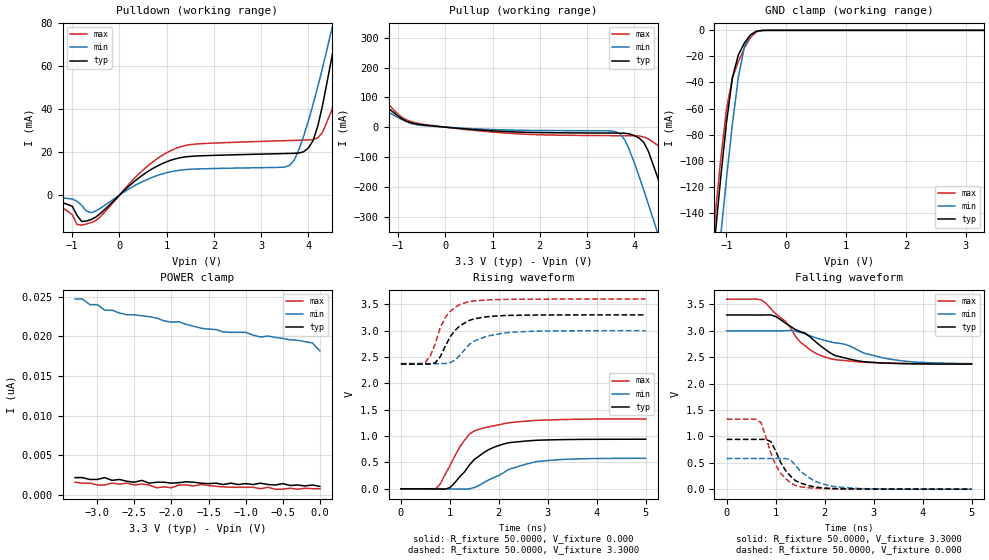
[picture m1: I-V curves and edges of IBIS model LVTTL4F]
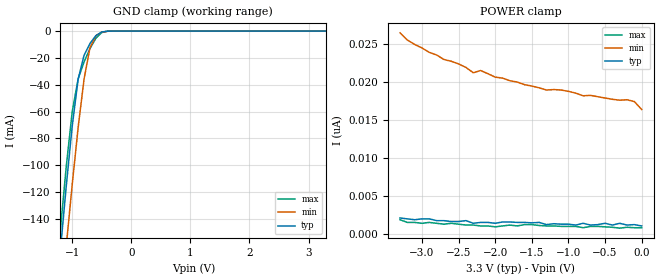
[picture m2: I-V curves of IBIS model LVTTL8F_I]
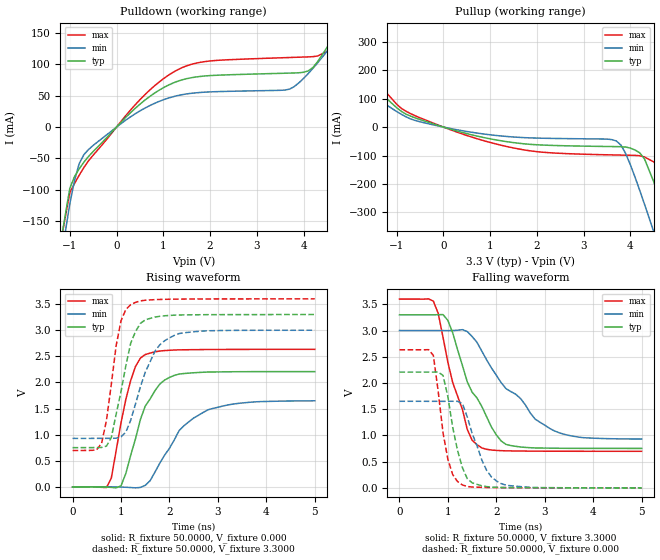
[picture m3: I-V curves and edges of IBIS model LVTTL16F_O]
| Xilinx Virtex IBIS File
[IBIS ver]   2.1
[File name]   virtex.ibs
[File Rev]   1.1
[Date]   Mar. 16, 2001
[Source]   Hspice simulations (23e: TT, SS, FF)
[Notes]   Xilinx IBIS model for Virtex I/O
   The package models are provided for BG432, BG352, BG256,
   BG560, HQ240, PQ240, CS144, TQ144, FG256, FG456, FG676
   and FG680 package types, with BG432 being selected as
   a default. Please make your own selection of the packages
   by commenting out the unused ones.
   COMMENTS: Models include process corners for MIN and MAX.
[Disclaimer] The data in this model is derived from SPICE simulations using
   modeling information extracted from the target process. While
   a great deal of care has been taken to provide information
   that is accurate, this model is considered preliminary as it
   has not been verified by actual silicon measurement. Treat the
   data in this model as preliminary until actual silicon
   verification is performed.
[Copyright]   Copyright 1998, Xilinx Inc., All rights reserved
|   Component Virtex
|   >>> Make Your Selection of the Package type Below <<<
[Component]   VIRTEX
[Manufacturer]   Xilinx Inc.
[Package]
| For Package type BG432:
| variable   typ   min   max
R_pkg   0.2500   0.1600   0.3500
L_pkg   4.9000nH   2.4000nH   7.4000nH
C_pkg   1.0500pF   0.8000pF   1.3000pF
| For Package type BG352:
| variable   typ   min   max
|R_pkg   0.2340   0.1640   0.3040
|L_pkg   6.5500nH   3.8000nH   9.3000nH
|C_pkg   1.0200pF   0.7300pF   1.3100pF
| For Package type BG256:
| variable   typ   min   max
|R_pkg   0.1780   0.1700   0.1850
|L_pkg   4.5000nH   2.3000nH   6.7000nH
|C_pkg   1.4500pF   1.2000pF   1.7000pF
| For Package type BG560:
| variable   typ   min   max
|R_pkg   0.2240   0.1480   0.3000
|L_pkg   5.4500nH   2.0000nH   8.9000nH
|C_pkg   1.0500pF   0.5000pF   1.6000pF
| For Package type HQ240:
| variable   typ   min   max
|R_pkg   0.208   0.202   0.215
|L_pkg   13.2nH   9.00nH   17.3nH
|C_pkg   2.25pF   2.00pF   2.50pF
| For Package type PQ240:
| variable   typ   min   max
|R_pkg   0.208   0.205   0.218
|L_pkg   18.9nH   11.9nH   25.8nH
|C_pkg   1.60pF   1.30pF   1.90pF
| For Package type CS144:
| variable   typ   min   max
|R_pkg   0.116   0.078   0.153
|L_pkg   3.55nH   1.5nH   5.60nH
|C_pkg   0.60pF   0.5pF   0.7pF
| For Package type TQ144:
| variable   typ   min   max
|R_pkg   0.118   0.112   0.124
|L_pkg   9.50nH   5.7nH   13.3nH
|C_pkg   0.95pF   0.8pF   1.1pF
| For Package type FG256:
| variable   typ   min   max
|R_pkg   0.141   0.095   0.187
|L_pkg   4.25nH   1.7nH   6.80nH
|C_pkg   0.75pF   0.60pF   0.90pF
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[Pin]  signal_name   model_name   R_pin   L_pin   C_pin
1   LVCMOS2   LVCMOS2
1I   LVCMOS2_I   LVCMOS2_I
1O   LVCMOS2_O   LVCMOS2_O
2   LVTTL2F   LVTTL2F
2I   LVTTL2F_I   LVTTL2F_I
2O   LVTTL2F_O   LVTTL2F_O
3   LVTTL4F   LVTTL4F
3I   LVTTL4F_I   LVTTL4F_I
3O   LVTTL4F_O   LVTTL4F_O
4   LVTTL6F   LVTTL6F
4I   LVTTL6F_I   LVTTL6F_I
4O   LVTTL6F_O   LVTTL6F_O
5   LVTTL8F   LVTTL8F
5I   LVTTL8F_I   LVTTL8F_I
5O   LVTTL8F_O   LVTTL8F_O
6   LVTTL12F   LVTTL12F
6I   LVTTL12F_I   LVTTL12F_I
6O   LVTTL12F_O   LVTTL12F_O
7   LVTTL16F   LVTTL16F
7I   LVTTL16F_I   LVTTL16F_I
7O   LVTTL16F_O   LVTTL16F_O
8   LVTTL24F   LVTTL24F
8I   LVTTL24F_I   LVTTL24F_I
8O   LVTTL24F_O   LVTTL24F_O
9   LVTTL2S   LVTTL2S
9I   LVTTL2S_I   LVTTL2S_I
9O   LVTTL2S_O   LVTTL2S_O
10   LVTTL4S   LVTTL4S
10I   LVTTL4S_I   LVTTL4S_I
10O   LVTTL4S_O   LVTTL4S_O
11   LVTTL6S   LVTTL6S
11I   LVTTL6S_I   LVTTL6S_I
11O   LVTTL6S_O   LVTTL6S_O
12   LVTTL8S   LVTTL8S
12I   LVTTL8S_I   LVTTL8S_I
12O   LVTTL8S_O   LVTTL8S_O
13   LVTTL12S   LVTTL12S
13I   LVTTL12S_I   LVTTL12S_I
13O   LVTTL12S_O   LVTTL12S_O
14   LVTTL16S   LVTTL16S
14I   LVTTL16S_I   LVTTL16S_I
14O   LVTTL16S_O   LVTTL16S_O
15   LVTTL24S   LVTTL24S
15I   LVTTL24S_I   LVTTL24S_I
15O   LVTTL24S_O   LVTTL24S_O
16   HSTL1   HSTL1
16I   HSTL1_I   HSTL1_I
16O   HSTL1_O   HSTL1_O
17   HSTL3   HSTL3
17I   HSTL3_I   HSTL3_I
17O   HSTL3_O   HSTL3_O
18   HSTL4   HSTL4
18I   HSTL4_I   HSTL4_I
18O   HSTL4_O   HSTL4_O
19   SSTL2C1   SSTL2C1
19I   SSTL2C1_I   SSTL2C1_I
19O   SSTL2C1_O   SSTL2C1_O
20   SSTL2C2   SSTL2C2
20I   SSTL2C2_I   SSTL2C2_I
20O   SSTL2C2_O   SSTL2C2_O
21   SSTL3C1   SSTL3C1
21I   SSTL3C1_I   SSTL3C1_I
21O   SSTL3C1_O   SSTL3C1_O
22   SSTL3C2   SSTL3C2
22I   SSTL3C2_I   SSTL3C2_I
22O   SSTL3C2_O   SSTL3C2_O
23   CTT   CTT
23I   CTT_I   CTT_I
23O   CTT_O   CTT_O
24   AGP   AGP
24I   AGP_I   AGP_I
24O   AGP_O   AGP_O
25   GTL   GTL
25I   GTL_I   GTL_I
25O   GTL_O   GTL_O
26   GTL-PLUS   GTL-PLUS
26I   GTL-PLUS_I   GTL-PLUS_I
26O   GTL-PLUS_O   GTL-PLUS_O
27   PCI33M5V   PCI33M5V
27I   PCI33M5V_I   PCI33M5V_I
27O   PCI33M5V_O   PCI33M5V_O
28   PCI33M3V   PCI33M3V
28I   PCI33M3V_I   PCI33M3V_I
28O   PCI33M3V_O   PCI33M3V_O
29   PCI66M3V   PCI66M3V
29I   PCI66M3V_I   PCI66M3V_I
29O   PCI66M3V_O   PCI66M3V_O
PGND   GND   GND
VCCO   VCCO   POWER
| Models and submodels in the file (87): LVCMOS2 (I/O), LVCMOS2_I (Input), LVCMOS2_O (Output), LVTTL2F (I/O), LVTTL2F_I (Input), LVTTL2F_O (Output), LVTTL4F (I/O), LVTTL4F_I (Input), LVTTL4F_O (Output), LVTTL6F (I/O), LVTTL6F_I (Input), LVTTL6F_O (Output), LVTTL8F (I/O), LVTTL8F_I (Input), LVTTL8F_O (Output), LVTTL12F (I/O), LVTTL12F_I (Input), LVTTL12F_O (Output), LVTTL16F (I/O), LVTTL16F_I (Input), LVTTL16F_O (Output), LVTTL24F (I/O), LVTTL24F_I (Input), LVTTL24F_O (Output), LVTTL2S (I/O), LVTTL2S_I (Input), LVTTL2S_O (Output), LVTTL4S (I/O), LVTTL4S_I (Input), LVTTL4S_O (Output), LVTTL6S (I/O), LVTTL6S_I (Input), LVTTL6S_O (Output), LVTTL8S (I/O), LVTTL8S_I (Input), LVTTL8S_O (Output), LVTTL12S (I/O), LVTTL12S_I (Input), LVTTL12S_O (Output), LVTTL16S (I/O), LVTTL16S_I (Input), LVTTL16S_O (Output), LVTTL24S (I/O), LVTTL24S_I (Input), LVTTL24S_O (Output), HSTL1 (I/O), HSTL1_I (Input), HSTL1_O (Output), HSTL3 (I/O), HSTL3_I (Input), HSTL3_O (Output), HSTL4 (I/O), HSTL4_I (Input), HSTL4_O (Output), SSTL2C1 (I/O), SSTL2C1_I (Input), SSTL2C1_O (Output), SSTL2C2 (I/O), SSTL2C2_I (Input), SSTL2C2_O (Output), SSTL3C1 (I/O), SSTL3C1_I (Input), SSTL3C1_O (Output), SSTL3C2 (I/O), SSTL3C2_I (Input), SSTL3C2_O (Output), CTT (I/O), CTT_I (Input), CTT_O (Output), AGP (I/O), AGP_I (Input), AGP_O (Output), GTL (I/O_open_drain), GTL_I (Input), GTL_O (Open_drain), GTL-PLUS (I/O_open_drain), GTL-PLUS_I (Input), GTL-PLUS_O (Open_drain), PCI33M5V (I/O), PCI33M5V_I (Input)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
|   Model LVTTL4F
[Model]   LVTTL4F
Model_type   I/O
Polarity   Non-Inverting
Enable   Active-Low
Vinl =   0.800V
Vinh =   2.000V
Vmeas =   1.4000V
Cref =  35.0000pF
Rref =   1.0000M
Vref =  0.000V
C_comp   6.5000pF   5.0000pF   8.0000pF
[Temperature Range]   27.0000   100.0000   0.000
[Voltage Range]   3.3000V   3.0000V   3.6000V
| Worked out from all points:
|   slope of the pulldown table from 0 to 0.495 V, typ, clamps not added: 52.7 ohm
|   slope of the pullup table from 0 to 0.495 V, typ, clamps not added: 72 ohm
|   GND clamp passes 1 mA (typ) near -0.51 V on its own axis
|   rising waveform, R_fixture 50.0000, V_fixture 0.000: 20-80 % time 649ps typ, 853ps min, 538ps max; typ from 0 V to 0.941 V
|   rising waveform, R_fixture 50.0000, V_fixture 3.3000: 20-80 % time 419ps typ, 526ps min, 353ps max; typ from 2.37 V to 3.3 V
|   falling waveform, R_fixture 50.0000, V_fixture 3.3000: 20-80 % time 914ps typ, 1.33ns min, 768ps max; typ from 3.3 V to 2.37 V
|   falling waveform, R_fixture 50.0000, V_fixture 0.000: 20-80 % time 386ps typ, 512ps min, 365ps max; typ from 0.943 V to 0.001 V
[Pulldown]
| voltage   I(typ)   I(min)   I(max)
-3.3V     0A         0A         -1mA
-1.5V     -1mA       -500uA     -1.2mA
-800mV    -12.23mA   -4.72mA    -13.9mA
-600mV    -11.34mA   -8.171mA   -12.78mA
1.2V      16.95mA    11.33mA    21.76mA
3.6V      19.37mA    13.78mA    25.36mA
3.8V      19.56mA    21.23mA    25.5mA
4.1V      25.44mA    42.35mA    25.81mA
4.5V      64.6mA     77.61mA    39.82mA
4.7V      89.71mA    97.03mA    64.96mA
4.9V      116.1mA    117.3mA    95.67mA
6.6V      348mA      295mA      376.7mA
[Pullup]
| voltage   I(typ)   I(min)   I(max)
-3.3V     354.4mA    271.9mA    429.9mA
-2.7V     272.8mA    207.8mA    331mA
-800mV    18.43mA    17.03mA    23.04mA
3.6V      -19.96mA   -15.22mA   -28.65mA
3.8V      -20.52mA   -43.41mA   -28.84mA
4.2V      -51mA      -211.2mA   -32.92mA
4.5V      -171.4mA   -357.8mA   -61.08mA
4.7V      -272mA     -457.9mA   -116mA
4.9V      -376.2mA   -559mA     -210.3mA
5.1V      -482.2mA   -660.7mA   -313.6mA
5.3V      -589.2mA   -762.8mA   -420.3mA
6.6V      -1.293A    -1.432A    -1.133A
[GND_clamp]
| voltage   I(typ)   I(min)   I(max)
-3.3V     -1.286A    -1.273A    -1.289A
-1.2V     -163.3mA   -206.7mA   -148.3mA
-1.1V     -115.2mA   -159.6mA   -101mA
-1V       -71.04mA   -114.2mA   -60.78mA
-900mV    -36.42mA   -71.86mA   -36.53mA
-800mV    -18.72mA   -35.86mA   -23.84mA
-700mV    -9.715mA   -12.62mA   -13.63mA
-600mV    -3.608mA   -3.649mA   -5.601mA
-500mV    -692.7uA   -854.2uA   -1.156mA
-400mV    -68.48uA   -138.7uA   -98.51uA
-300mV    -4.365uA   -16.73uA   -4.597uA
3.3V      1.106nA    19.44nA    698.5pA
[POWER_clamp]
| voltage   I(typ)   I(min)   I(max)
-3.3V     2.212nA    24.68nA    1.63nA
-3.2V     2.212nA    24.68nA    1.513nA
-3.1V     1.979nA    23.98nA    1.513nA
-3V       1.979nA    23.98nA    1.281nA
-2.9V     2.212nA    23.28nA    1.281nA
-2.6V     1.746nA    22.7nA     1.513nA
-2.2V     1.63nA     22.29nA    931.3pA
-1.6V     1.513nA    21.01nA    1.339nA
-1V       1.455nA    20.49nA    989.5pA
-800mV    1.513nA    19.91nA    814.9pA
-100mV    1.281nA    19.15nA    814.9pA
0V        1.106nA    18.16nA    814.9pA
[Ramp]
| variable   typ   min   max
dV/dt_r   0.5647/0.6500n   0.3480/0.8497n   0.7950/0.5579n
dV/dt_f   0.5586/0.9517n   0.3726/1.3252n   0.7338/0.7688n
R_load = 50.0000
[Rising Waveform]
R_fixture = 50.0000
V_fixture = 0.000
| time   V(typ)   V(min)   V(max)
0s        0V         0V         0V
700ps     -2.021mV   226.2uV    -4.415mV
800ps     -4.588mV   188uV      85.45mV
1ns       21.52mV    -1.672mV   434.2mV
1.3ns     321.5mV    -6.047mV   921.4mV
1.5ns     557.2mV    23.94mV    1.1V
1.7ns     692mV      121.2mV    1.157V
2.2ns     873.5mV    365.6mV    1.253V
2.8ns     922.2mV    519.7mV    1.3V
5ns       941.2mV    580mV      1.325V
[Rising Waveform]
R_fixture = 50.0000
V_fixture = 3.3000
V_fixture_min = 3.0000
V_fixture_max = 3.6000
| time   V(typ)   V(min)   V(max)
0s        2.365V     2.374V     2.375V
500ps     2.365V     2.374V     2.397V
700ps     2.39V      2.374V     2.744V
800ps     2.499V     2.374V     3.043V
900ps     2.691V     2.377V     3.237V
1.1ns     3V         2.437V     3.439V
1.4ns     3.195V     2.74V      3.551V
1.7ns     3.256V     2.876V     3.579V
2.2ns     3.289V     2.966V     3.594V
5ns       3.299V     2.999V     3.599V
[Falling Waveform]
R_fixture = 50.0000
V_fixture = 3.3000
V_fixture_min = 3.0000
V_fixture_max = 3.6000
| time   V(typ)   V(min)   V(max)
0s        3.3V       3V         3.6V
700ps     3.299V     3V         3.587V
1ns       3.272V     2.999V     3.325V
1.2ns     3.145V     3.002V     3.18V
1.5ns     2.987V     2.97V      2.789V
1.8ns     2.807V     2.874V     2.584V
2.1ns     2.591V     2.795V     2.477V
2.7ns     2.429V     2.625V     2.411V
3.4ns     2.384V     2.454V     2.388V
5ns       2.369V     2.379V     2.377V
[Falling Waveform]
R_fixture = 50.0000
V_fixture = 0.000
| time   V(typ)   V(min)   V(max)
0s        943.3mV    581.6mV    1.327V
600ps     943.4mV    581.6mV    1.325V
700ps     943.7mV    581.6mV    1.262V
900ps     903.3mV    581.6mV    689.3mV
1ns       728.3mV    581.8mV    460.1mV
1.2ns     357.9mV    581.3mV    201.4mV
1.4ns     164mV      456.6mV    71.6mV
1.8ns     43.47mV    155.2mV    18.74mV
2.2ns     11.27mV    47.74mV    7.191mV
5ns       636.3uV    446.4uV    717.8uV
|   Model LVTTL8F_I
[Model]   LVTTL8F_I
Model_type   Input
Polarity   Non-Inverting
Vinl =   0.800V
Vinh =   2.000V
C_comp   6.5000pF   5.0000pF   8.0000pF
[Temperature Range]   27.0000   100.0000   0.000
[Voltage Range]   3.3000V   3.0000V   3.6000V
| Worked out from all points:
|   GND clamp passes 1 mA (typ) near -0.51 V on its own axis
[GND_clamp]
| voltage   I(typ)   I(min)   I(max)
-3.3V     -1.286A    -1.273A    -1.29A
-1.3V     -213.2mA   -255.1mA   -198mA
-1.2V     -163mA     -206.8mA   -147.7mA
-1.1V     -114.8mA   -159.6mA   -100.3mA
-1V       -70.57mA   -114.1mA   -59.86mA
-900mV    -35.79mA   -71.75mA   -35.46mA
-800mV    -18.04mA   -35.69mA   -22.98mA
-700mV    -9.256mA   -12.38mA   -13.06mA
-600mV    -3.388mA   -3.468mA   -5.299mA
-500mV    -637.4uA   -792.4uA   -1.07mA
-300mV    -3.973uA   -15.32uA   -4.185uA
3.3V      1.048nA    17.58nA    698.5pA
[POWER_clamp]
| voltage   I(typ)   I(min)   I(max)
-3.3V     2.095nA    26.43nA    1.863nA
-3.1V     1.863nA    24.91nA    1.513nA
-2.7V     1.746nA    22.93nA    1.281nA
-2.4V     1.746nA    21.89nA    1.164nA
-2.3V     1.397nA    21.19nA    1.164nA
-2.2V     1.513nA    21.48nA    1.048nA
-2V       1.397nA    20.61nA    931.3pA
-1.4V     1.513nA    19.21nA    1.106nA
-1.3V     1.222nA    18.92nA    1.048nA
-200mV    1.164nA    17.64nA    873.1pA
-100mV    1.222nA    17.4nA     814.9pA
0V        1.048nA    16.36nA    814.9pA
|   Model LVTTL16F_O
[Model]   LVTTL16F_O
Model_type   Output
Polarity   Non-Inverting
Vmeas =   1.4000V
Cref =  35.0000pF
Rref =   1.0000M
Vref =  0.000V
C_comp   6.5000pF   5.0000pF   8.0000pF
[Temperature Range]   27.0000   100.0000   0.000
[Voltage Range]   3.3000V   3.0000V   3.6000V
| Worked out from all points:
|   slope of the pulldown table from 0 to 0.495 V, typ, clamps not added: 13.7 ohm
|   slope of the pullup table from 0 to 0.495 V, typ, clamps not added: 21.7 ohm
|   rising waveform, R_fixture 50.0000, V_fixture 0.000: 20-80 % time 500ps typ, 772ps min, 357ps max; typ from 0 V to 2.21 V
|   rising waveform, R_fixture 50.0000, V_fixture 3.3000: 20-80 % time 348ps typ, 474ps min, 266ps max; typ from 0.751 V to 3.3 V
|   falling waveform, R_fixture 50.0000, V_fixture 3.3000: 20-80 % time 696ps typ, 1.06ns min, 490ps max; typ from 3.3 V to 0.752 V
|   falling waveform, R_fixture 50.0000, V_fixture 0.000: 20-80 % time 289ps typ, 392ps min, 245ps max; typ from 2.21 V to 0 V
[Pulldown]
| voltage   I(typ)   I(min)   I(max)
-3.3V     -1.282A    -1.27A     -1.284A
-1.5V     -319.5mA   -354.4mA   -307.2mA
-1V       -97.76mA   -122.6mA   -104.7mA
-800mV    -66.75mA   -58.46mA   -76.88mA
-600mV    -46.92mA   -35.82mA   -53.89mA
600mV     42.55mA    29.94mA    51.16mA
1.4V      75.27mA    51.64mA    94.7mA
3.7V      86.04mA    60.44mA    110.9mA
4.1V      89.48mA    85.22mA    111.9mA
4.5V      126.6mA    120.5mA    120.3mA
4.9V      177.6mA    159.9mA    174.2mA
6.6V      407.8mA    336.3mA    452.6mA
[Pullup]
| voltage   I(typ)   I(min)   I(max)
-3.3V     413.8mA    317.9mA    498.5mA
-2.9V     356.6mA    273mA      429.3mA
-2.5V     297.6mA    226.1mA    358.6mA
-600mV    31.98mA    22.96mA    39.44mA
1.5V      -54.66mA   -34.94mA   -73.46mA
3.7V      -68.75mA   -48.9mA    -98.25mA
3.9V      -70.27mA   -93.43mA   -98.9mA
4.2V      -90.62mA   -222.7mA   -100.8mA
4.5V      -192.3mA   -368.3mA   -122.6mA
4.9V      -393.7mA   -569.2mA   -241mA
5.1V      -499.3mA   -670.9mA   -340.5mA
6.6V      -1.31A     -1.442A    -1.157A
[Ramp]
| variable   typ   min   max
dV/dt_r   1.3242/0.4985n   0.9888/0.7729n   1.5792/0.3516n
dV/dt_f   1.5287/0.6938n   1.2413/1.0975n   1.7416/0.4965n
R_load = 50.0000
[Rising Waveform]
R_fixture = 50.0000
V_fixture = 0.000
| time   V(typ)   V(min)   V(max)
0s        0V         0V         0V
700ps     -3.795mV   862.2uV    -13.55mV
800ps     -9.498mV   979.2uV    167.9mV
1ns       20.18mV    -3.712mV   1.226V
1.3ns     923.5mV    -18.43mV   2.307V
1.5ns     1.546V     29.14mV    2.533V
2ns       2.095V     737.9mV    2.615V
2.3ns     2.17V      1.171V     2.624V
2.8ns     2.199V     1.477V     2.629V
5ns       2.207V     1.648V     2.632V
[Rising Waveform]
R_fixture = 50.0000
V_fixture = 3.3000
V_fixture_min = 3.0000
V_fixture_max = 3.6000
| time   V(typ)   V(min)   V(max)
0s        751.2mV    928.2mV    696.8mV
600ps     755.2mV    928.8mV    836.4mV
800ps     943.5mV    928.5mV    1.963V
900ps     1.393V     932.2mV    2.704V
1ns       1.821V     959.1mV    3.179V
1.2ns     2.748V     1.276V     3.488V
1.4ns     3.129V     1.913V     3.56V
1.7ns     3.251V     2.595V     3.584V
2.1ns     3.287V     2.9V       3.593V
5ns       3.299V     2.999V     3.599V
[Falling Waveform]
R_fixture = 50.0000
V_fixture = 3.3000
V_fixture_min = 3.0000
V_fixture_max = 3.6000
| time   V(typ)   V(min)   V(max)
0s        3.3V       3V         3.6V
700ps     3.299V     3V         3.562V
800ps     3.303V     3V         3.329V
1ns       3.193V     2.999V     2.395V
1.4ns     2.023V     2.981V     1.116V
1.7ns     1.554V     2.608V     761.8mV
2ns       1.01V      2.148V     714.3mV
2.2ns     828.5mV    1.892V     706mV
3.1ns     757.3mV    1.135V     699.1mV
5ns       752.1mV    931.2mV    697.4mV
[Falling Waveform]
R_fixture = 50.0000
V_fixture = 0.000
| time   V(typ)   V(min)   V(max)
0s        2.208V     1.651V     2.633V
700ps     2.208V     1.651V     2.528V
900ps     2.144V     1.65V      1.05V
1ns       1.74V      1.651V     545.6mV
1.1ns     1.151V     1.651V     251.9mV
1.3ns     385.6mV    1.607V     55.11mV
1.5ns     96.7mV     1.042V     16.4mV
1.8ns     23.75mV    334.2mV    8.086mV
2.1ns     8.195mV    81.18mV    4.432mV
5ns       477.8uV    527.6uV    435.5uV
